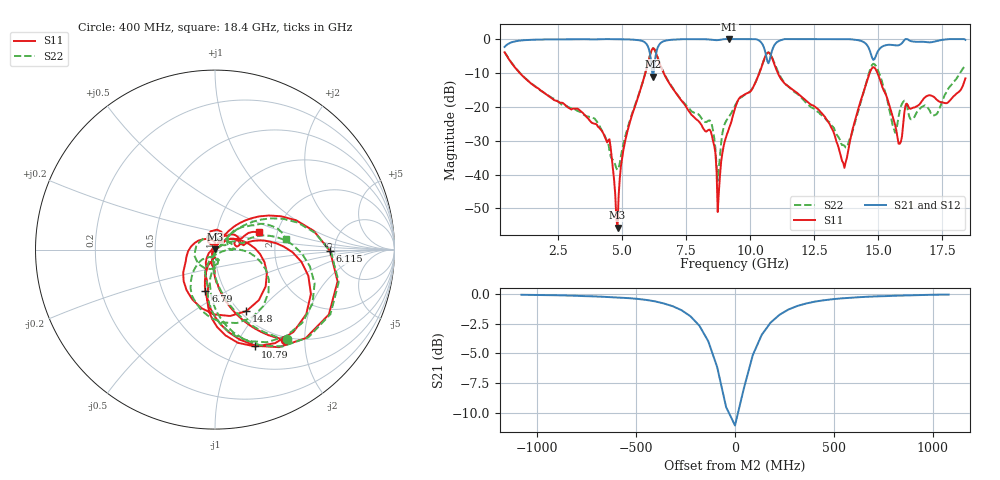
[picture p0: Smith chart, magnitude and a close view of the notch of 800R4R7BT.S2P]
!  American Technical Ceramics  Date:  10/25/10
!  One Norden Lane
!  Huntington Station,  NY.  11746-2102
!  Tel:  (631) 622-4700  Fax:  (631) 622-4748
!  Part Number  800R4R7BT.TXT  Mounting Orientation: Horizontal
!  Description: Ultra Low ESR Microwave Capacitor
!  Application: Coupling, Bypass, Tuning, DC Block, Filters, Matching
# GHZ S DB R 50
! Freq  |S11|  S11 Ph  |S21|  S21 Ph  |S12|  S12 Ph  |S22|  S22 Ph
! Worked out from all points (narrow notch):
!   401 points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, 400 MHz to 18.4 GHz, reference 50 ohm
!   highest |S21| = -0.01 dB at 9.175 GHz (marker M1); lowest = -11.1 dB at 6.205 GHz (marker M2)
!   notch at M2: 11.0 dB deep, 185 MHz wide at half that depth
!   lowest |S11| = -55.7 dB at 4.81 GHz (marker M3), VSWR 1.00, Z = 50 + j0.16 ohm
!   |S11| at or under -10 dB: 990 MHz to 5.899 GHz (4.909 GHz wide, 143 % of centre); 6.612 GHz to 10.35 GHz (3.742 GHz wide, 44.1 % of centre); 11.07 GHz to 14.66 GHz (3.592 GHz wide, 27.9 % of centre)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
!   |S22| runs from -41.9 to -2.7 dB; largest |S21 - S12| = 0.0068
!   S11 on the Smith chart (normalised r, x): 400 MHz: 0.95, -1.62; 6.115 GHz: 4.57, -0.12; 6.79 GHz: 0.81, -0.40; 10.79 GHz: 0.74, -1.21; 14.8 GHz: 1.07, -0.86; 18.4 GHz: 1.60, +0.34
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0.4  -3.91 -52.0  -2.33 38.1  -2.37 38.1  -3.85 -51.1
3.415  -21.53 -102.3  -0.04 -10.3  -0.07 -10.2  -21.97 -96.0
4.45  -30.02 -104.7  -0.02 -17.7  -0.04 -17.6  -30.72 -100.2
4.81  -55.69 103.6  -0.06 -20.4  -0.07 -20.2  -38.64 -24.7
6.115  -3.86 -0.7  -6.17 -57.1  -6.18 -57.0  -3.77 -1.4
6.205  -2.73 -29.7  -11.07 -14.1  -11.08 -13.8  -2.65 -29.3
6.43  -6.63 -80.6  -1.76 1.4  -1.76 1.6  -6.52 -77.5
6.79  -12.52 -103.1  -0.33 -13.4  -0.32 -13.2  -12.38 -95.7
8.455  -27.31 -99.6  -0.17 -30.9  -0.14 -30.6  -24.41 -79.3
8.77  -45.03 16.2  -0.28 -30.5  -0.25 -30.3  -38.11 14.4
9.175  -26.18 35.8  -0.01 -33.1  -0.01 -32.8  -22.84 23.8
9.4  -20.46 37.9  -0.01 -34.4  -0.01 -34.2  -19.68 25.2
10.39  -9.27 5.8  -0.74 -57.7  -0.70 -57.5  -9.16 11.6
10.795  -4.67 -67.5  -4.88 -19.7  -4.87 -19.7  -4.57 -60.9
12.415  -19.53 -116.6  -0.01 -46.3  -0.01 -46.4  -20.31 -115.1
13.675  -38.02 138.7  -0.01 -57.6  -0.01 -57.7  -31.51 -70.8
14.8  -8.30 -62.9  -6.13 -63.5  -6.09 -63.6  -7.31 -61.4
15.43  -19.45 152.5  -1.68 -50.3  -1.65 -50.6  -20.81 -142.4
15.835  -30.93 107.4  -1.70 -46.9  -1.67 -47.1  -21.25 -81.7
16.105  -19.06 84.5  -0.01 -52.4  -0.01 -52.5  -19.44 165.7
17.23  -17.54 9.4  -0.65 -56.3  -0.62 -56.6  -22.36 23.2
18.4  -11.62 21.8  -0.24 -77.4  -0.21 -77.7  -7.98 8.8
